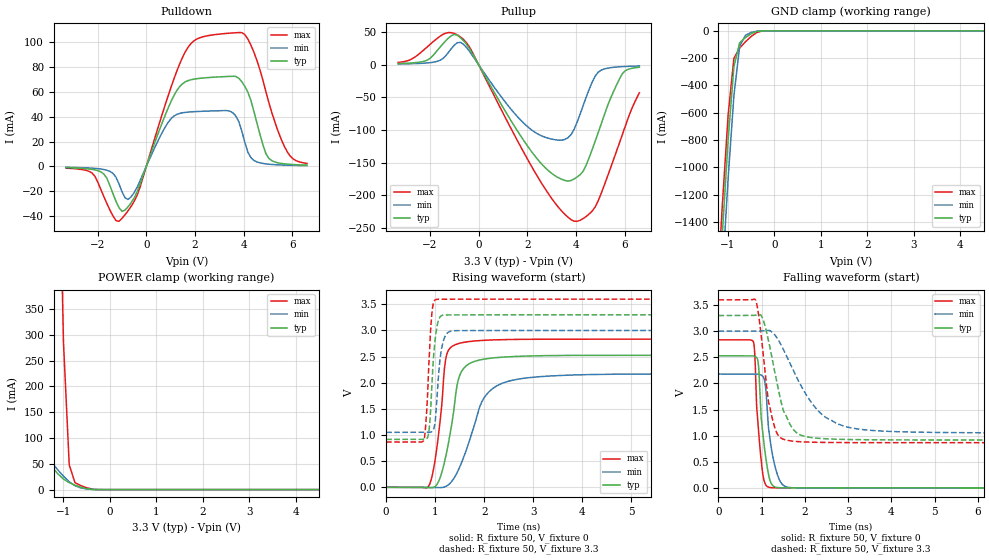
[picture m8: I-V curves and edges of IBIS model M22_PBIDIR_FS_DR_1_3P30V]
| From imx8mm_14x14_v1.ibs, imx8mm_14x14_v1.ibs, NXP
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[Model] M22_PBIDIR_FS_DR_1_3P30V
Model_type I/O
Vinl  =  0.54
Vinh  =  1.26
Vmeas =  0.9
| Capacitance   typ   min   max
C_comp   2.08161232969e-12   2.03493647009e-12   2.16777276051e-12
| Variables   typ   min   max
[GND Clamp Reference]   0   0   0
[POWER Clamp Reference]   3.3   3   3.6
[Pulldown Reference]   0   0   0
[Pullup Reference]   3.3   3   3.6
[Temperature Range]   25   125   -40
[Voltage Range]   3.3   3   3.6
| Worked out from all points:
|   slope of the pulldown table from 0 to 0.495 V, typ, clamps not added: 18.4 ohm
|   slope of the pullup table from 0 to 0.495 V, typ, clamps not added: 15.2 ohm
|   GND clamp passes 1 mA (typ) near -0.28 V on its own axis
|   POWER clamp passes 1 mA (typ) near -0.44 V on its own axis
|   falling waveform, R_fixture 50, V_fixture 0: 20-80 % time 155ps typ, 191ps min, 128ps max; typ from 2.53 V to 0 V
|   falling waveform, R_fixture 50, V_fixture 3.3: 20-80 % time 401ps typ, 823ps min, 253ps max; typ from 3.3 V to 0.916 V
|   rising waveform, R_fixture 50, V_fixture 0: 20-80 % time 266ps typ, 498ps min, 183ps max; typ from 0 V to 2.53 V
|   rising waveform, R_fixture 50, V_fixture 3.3: 20-80 % time 96.7ps typ, 105ps min, 86.4ps max; typ from 0.916 V to 3.3 V
[GND Clamp]
| Voltage   I(typ)   I(min)   I(max)
-3.3V     -15.63A    -15.86A    -15.46A
-1.241V   -2.232A    -2.527A    -2.015A
-1.117V   -1.487A    -1.785A    -1.276A
-993.1mV  -798.9mA   -1.083A    -616.8mA
-869mV    -263.4mA   -475.6mA   -200.8mA
-744.8mV  -87.36mA   -112.1mA   -126.1mA
-620.7mV  -49.17mA   -33.01mA   -80.34mA
-496.6mV  -20.8mA    -11.81mA   -40.7mA
-372.4mV  -3.877mA   -2.002mA   -11.64mA
-248.3mV  -117.5uA   -105.1uA   -542.9uA
6.6V      0A         0A         0A
[POWER Clamp]
| Voltage   I(typ)   I(min)   I(max)
-3.3V     11.6A      9.427A     14.09A
-1.862V   2.37A      558.5mA    4.855A
-1.738V   1.676A     202.6mA    4.157A
-1.614V   1.03A      99.77mA    3.468A
-1.49V    451mA      80.49mA    2.786A
-1.366V   91.11mA    66.06mA    2.111A
-1.241V   43.77mA    52.06mA    1.45A
-1.117V   30.97mA    38.55mA    817.5mA
-993.1mV  20.41mA    25.92mA    286.6mA
-869mV    13.37mA    15.08mA    47.85mA
-744.8mV  8.524mA    7.507mA    13.32mA
6.6V      0A         0A         0A
[Pulldown]
| Voltage   I(typ)   I(min)   I(max)
-3.3V     -1.009mA   -698.4uA   -1.399mA
-2.234V   -2.355mA   -1.393mA   -5.168mA
-1.738V   -6.137mA   -2.501mA   -24.35mA
-1.117V   -33.17mA   -14.12mA   -44.04mA
-620.7mV  -29.12mA   -24.39mA   -31.98mA
910.3mV   47.41mA    35.65mA    57.4mA
1.707V    68.78mA    43.57mA    95.36mA
3.797V    70.85mA    36.06mA    107.4mA
4.293V    53.17mA    7.074mA    97.48mA
5.038V    6.305mA    1.771mA    50.87mA
5.783V    1.853mA    982.8uA    11.9mA
6.6V      1.043mA    656.1uA    2.434mA
[Pullup]
| Voltage   I(typ)   I(min)   I(max)
-3.3V     1.756mA    1.099mA    3.431mA
-2.11V    6.905mA    2.684mA    27.15mA
-1.366V   35.93mA    12.91mA    48.11mA
-993.1mV  46.43mA    30.07mA    47.78mA
-620.7mV  36.85mA    31.24mA    38.64mA
2.162V    -132.4mA   -99.46mA   -154.8mA
3.3V      -173.4mA   -115.6mA   -219.3mA
3.921V    -175mA     -98.98mA   -239.5mA
4.293V    -163mA     -62.52mA   -235.6mA
4.914V    -103.6mA   -11.38mA   -208mA
5.907V    -13.53mA   -2.968mA   -106.5mA
6.6V      -3.952mA   -1.982mA   -43.03mA
[Ramp]
dV/dt_r   1.51721/0.266508n  1.30726/0.498444n  1.70108/0.182561n
dV/dt_f   1.43022/0.400979n  1.16928/0.822733n  1.64106/0.253483n
R_load = 50
[Falling Waveform]
R_fixture = 50
V_fixture = 0
V_fixture_min = 0
V_fixture_max = 0
| Time   V(typ)   V(min)   V(max)
0s        2.529V     2.18V      2.835V
809.1ps   2.526V     2.18V      2.793V
919.5ps   2.389V     2.178V     1.167V
1.022ns   1.068V     2.138V     280.4mV
1.088ns   611.5mV    1.937V     64.74mV
1.16ns    244.3mV    1.136V     12.69mV
1.293ns   21.83mV    459.3mV    1.126mV
1.48ns    1.462mV    63.76mV    986.7uV
1.847ns   473.6uV    826.4uV    711.7uV
333.3ns   925.6nV    1.69uV     3.322uV
[Falling Waveform]
R_fixture = 50
V_fixture = 3.3
V_fixture_min = 3
V_fixture_max = 3.6
| Time   V(typ)   V(min)   V(max)
0s        3.3V       3V         3.6V
864.9ps   3.304V     3V         3.586V
1.002ns   3.279V     3.003V     2.816V
1.153ns   2.835V     3.018V     1.667V
1.39ns    1.866V     2.824V     997.7mV
1.779ns   1.076V     2.167V     889.8mV
2.602ns   935.2mV    1.299V     868.5mV
3.721ns   919.7mV    1.09V      865.4mV
8.095ns   916.3mV    1.052V     864.9mV
333.3ns   916.3mV    1.051V     864.9mV
[Rising Waveform]
R_fixture = 50
V_fixture = 0
V_fixture_min = 0
V_fixture_max = 0
| Time   V(typ)   V(min)   V(max)
0s        925.5nV    1.69uV     3.322uV
886.4ps   -7.876mV   -540uV     59.56mV
1.051ns   79.31mV    -8.181mV   876.9mV
1.206ns   552.3mV    12.1mV     2.412V
1.299ns   996.5mV    73.02mV    2.659V
1.453ns   1.985V     292.5mV    2.744V
1.587ns   2.282V     590.6mV    2.774V
2.017ns   2.455V     1.739V     2.813V
2.704ns   2.506V     2.071V     2.83V
333.3ns   2.529V     2.179V     2.835V
[Rising Waveform]
R_fixture = 50
V_fixture = 3.3
V_fixture_min = 3
V_fixture_max = 3.6
| Time   V(typ)   V(min)   V(max)
0s        916.3mV    1.051V     864.9mV
770ps     916.3mV    1.051V     906.2mV
828.8ps   934.9mV    1.051V     1.493V
870.3ps   1.063V     1.051V     2.361V
938.4ps   2.079V     1.071V     3.381V
1.002ns   2.856V     1.282V     3.588V
1.09ns    3.248V     2.384V     3.598V
1.245ns   3.298V     2.949V     3.599V
1.721ns   3.299V     2.999V     3.599V
333.3ns   3.3V       3V         3.6V
[Add Submodel]
| Submodel Name Mode
M22_PBIDIR_FS_DR_1_3P30V_T All
